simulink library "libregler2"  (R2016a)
settings: Solver=ode45  SolverMode=SingleTasking  StartTime=0.0  StopTime=10.0  RelTol=1e-3
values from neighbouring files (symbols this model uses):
  b0 = 5e3    (= 5000)    [init_epidemie.m]
  g = 9.81    [init_pendelStange.m]
  l = 1    [init_pendelStange.m]    (also in sfun_pendelstangeanim.m = block.DialogPrm(2).Data)
  M = block.DialogPrm(1).Data    [sfun_inferenz.m]
  om0 = 0    [init_pendelStange.m]
  T = 2    [fourierrechteck.m]
undefined symbols (not defined in the file or in its folder): D, h, Kd, Ki, Kp, mk, ml, n, offset, w, x0
libraries: libregler2 x22, simulink x1

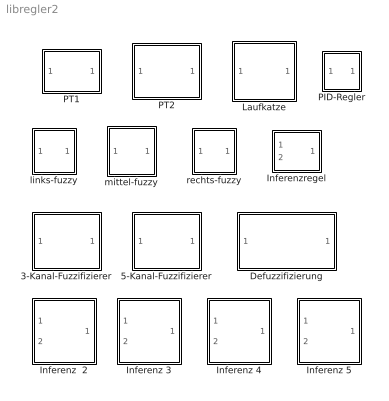
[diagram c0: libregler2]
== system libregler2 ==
  3-Kanal-Fuzzifizierer : Subsystem
  5-Kanal-Fuzzifizierer : Subsystem
  Defuzzifizierung : Subsystem
  Inferenz  2 : Subsystem
  Inferenz 3 : Subsystem
  Inferenz 4 : Subsystem
  Inferenz 5 : Subsystem
  Inferenzregel : Subsystem
  Laufkatze : Subsystem
  PID-Regler : Subsystem
  PT1 : Subsystem
  PT2 : Subsystem
  links-fuzzy : Subsystem
  mittel-fuzzy : Subsystem
  rechts-fuzzy : Subsystem

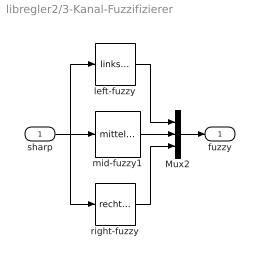
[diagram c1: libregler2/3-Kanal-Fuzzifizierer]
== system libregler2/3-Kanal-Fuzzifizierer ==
  sharp : Inport
  Mux2 : Mux  Inputs=3
  left-fuzzy : libregler2/links-fuzzy  SystemSampleTime=-1  x0=offset-w  w=w
  mid-fuzzy1 : libregler2/mittel-fuzzy  SystemSampleTime=-1  x0=offset  w=w
  right-fuzzy : libregler2/rechts-fuzzy  SystemSampleTime=-1  x0=offset+w  w=w
  fuzzy : Outport
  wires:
  sharp/1 -> right-fuzzy/1, left-fuzzy/1, mid-fuzzy1/1
  Mux2/1 -> fuzzy/1
  mid-fuzzy1/1 -> Mux2/2
  right-fuzzy/1 -> Mux2/3
  left-fuzzy/1 -> Mux2/1

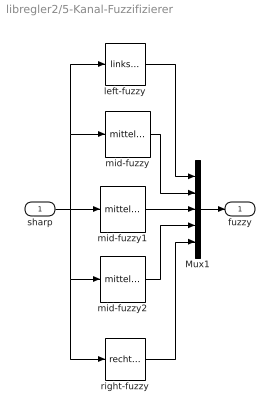
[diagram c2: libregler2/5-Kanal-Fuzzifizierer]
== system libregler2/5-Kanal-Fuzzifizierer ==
  sharp : Inport
  Mux1 : Mux  Inputs=5
  left-fuzzy : libregler2/links-fuzzy  SystemSampleTime=-1  x0=offset-2*w  w=w
  mid-fuzzy : libregler2/mittel-fuzzy  SystemSampleTime=-1  x0=offset-w  w=w
  mid-fuzzy1 : libregler2/mittel-fuzzy  SystemSampleTime=-1  x0=offset  w=w
  mid-fuzzy2 : libregler2/mittel-fuzzy  SystemSampleTime=-1  x0=offset+w  w=w
  right-fuzzy : libregler2/rechts-fuzzy  SystemSampleTime=-1  x0=offset+2*w  w=w
  fuzzy : Outport
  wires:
  Mux1/1 -> fuzzy/1
  sharp/1 -> mid-fuzzy/1, left-fuzzy/1, mid-fuzzy2/1, right-fuzzy/1, mid-fuzzy1/1
  right-fuzzy/1 -> Mux1/5
  mid-fuzzy2/1 -> Mux1/4
  mid-fuzzy1/1 -> Mux1/3
  mid-fuzzy/1 -> Mux1/2
  left-fuzzy/1 -> Mux1/1

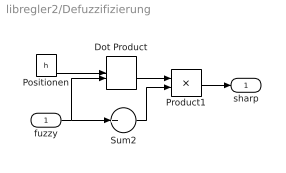
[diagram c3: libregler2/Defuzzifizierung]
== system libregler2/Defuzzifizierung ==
  fuzzy : Inport
  Dot Product : DotProduct
  Positionen : Constant  Value=h
  Product1 : Product  Inputs=*/
  Sum2 : Sum  Inputs=+
  sharp : Outport
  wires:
  Dot Product/1 -> Product1/1
  fuzzy/1 -> Sum2/1, Dot Product/2
  Positionen/1 -> Dot Product/1
  Sum2/1 -> Product1/2
  Product1/1 -> sharp/1

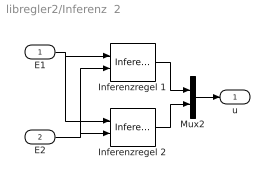
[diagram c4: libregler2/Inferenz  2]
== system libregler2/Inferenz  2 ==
  E1 : Inport
  E2 : Inport  Port=2
  Inferenzregel 1 : libregler2/Inferenzregel  SystemSampleTime=-1  M=M  n=1
  Inferenzregel 2 : libregler2/Inferenzregel  SystemSampleTime=-1  M=M  n=2
  Mux2 : Mux  Inputs=2
  u : Outport
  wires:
  E2/1 -> Inferenzregel 2/2, Inferenzregel 1/2
  E1/1 -> Inferenzregel 2/1, Inferenzregel 1/1
  Inferenzregel 1/1 -> Mux2/1
  Mux2/1 -> u/1
  Inferenzregel 2/1 -> Mux2/2

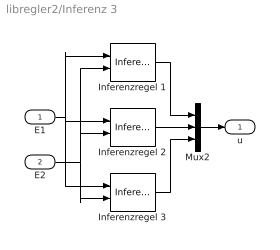
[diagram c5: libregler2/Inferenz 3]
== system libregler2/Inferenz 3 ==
  note: .
  E1 : Inport
  E2 : Inport  Port=2
  Inferenzregel 1 : libregler2/Inferenzregel  SystemSampleTime=-1  M=M  n=1
  Inferenzregel 2 : libregler2/Inferenzregel  SystemSampleTime=-1  M=M  n=2
  Inferenzregel 3 : libregler2/Inferenzregel  SystemSampleTime=-1  M=M  n=3
  Mux2 : Mux  Inputs=3
  u : Outport
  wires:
  E2/1 -> Inferenzregel 3/2, Inferenzregel 1/2, Inferenzregel 2/2
  E1/1 -> Inferenzregel 1/1, Inferenzregel 2/1, Inferenzregel 3/1
  Inferenzregel 3/1 -> Mux2/3
  Inferenzregel 1/1 -> Mux2/1
  Mux2/1 -> u/1
  Inferenzregel 2/1 -> Mux2/2

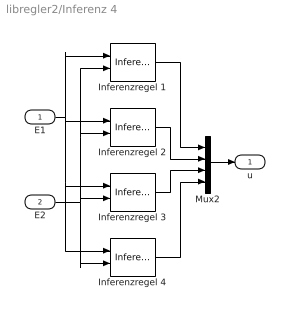
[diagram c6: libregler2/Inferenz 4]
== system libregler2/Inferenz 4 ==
  E1 : Inport
  E2 : Inport  Port=2
  Inferenzregel 1 : libregler2/Inferenzregel  SystemSampleTime=-1  M=M  n=1
  Inferenzregel 2 : libregler2/Inferenzregel  SystemSampleTime=-1  M=M  n=2
  Inferenzregel 3 : libregler2/Inferenzregel  SystemSampleTime=-1  M=M  n=3
  Inferenzregel 4 : libregler2/Inferenzregel  SystemSampleTime=-1  M=M  n=4
  Mux2 : Mux
  u : Outport
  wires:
  E2/1 -> Inferenzregel 2/2, Inferenzregel 1/2, Inferenzregel 3/2, Inferenzregel 4/2
  E1/1 -> Inferenzregel 2/1, Inferenzregel 1/1, Inferenzregel 3/1, Inferenzregel 4/1
  Inferenzregel 3/1 -> Mux2/3
  Inferenzregel 1/1 -> Mux2/1
  Mux2/1 -> u/1
  Inferenzregel 2/1 -> Mux2/2
  Inferenzregel 4/1 -> Mux2/4

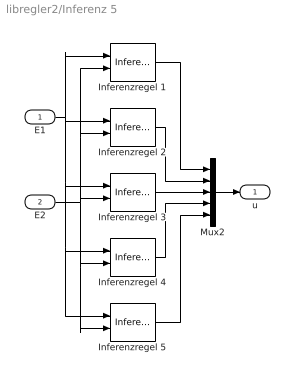
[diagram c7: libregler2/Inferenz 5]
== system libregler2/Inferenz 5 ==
  E1 : Inport
  E2 : Inport  Port=2
  Inferenzregel 1 : libregler2/Inferenzregel  SystemSampleTime=-1  M=M  n=1
  Inferenzregel 2 : libregler2/Inferenzregel  SystemSampleTime=-1  M=M  n=2
  Inferenzregel 3 : libregler2/Inferenzregel  SystemSampleTime=-1  M=M  n=3
  Inferenzregel 4 : libregler2/Inferenzregel  SystemSampleTime=-1  M=M  n=4
  Inferenzregel 5 : libregler2/Inferenzregel  SystemSampleTime=-1  M=M  n=5
  Mux2 : Mux  Inputs=5
  u : Outport
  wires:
  E2/1 -> Inferenzregel 3/2, Inferenzregel 4/2, Inferenzregel 5/2, Inferenzregel 1/2, Inferenzregel 2/2
  E1/1 -> Inferenzregel 3/1, Inferenzregel 4/1, Inferenzregel 5/1, Inferenzregel 1/1, Inferenzregel 2/1
  Inferenzregel 3/1 -> Mux2/3
  Inferenzregel 1/1 -> Mux2/1
  Mux2/1 -> u/1
  Inferenzregel 2/1 -> Mux2/2
  Inferenzregel 4/1 -> Mux2/4
  Inferenzregel 5/1 -> Mux2/5

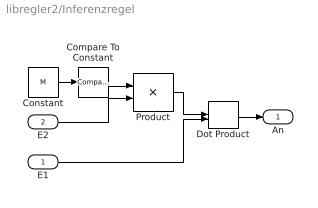
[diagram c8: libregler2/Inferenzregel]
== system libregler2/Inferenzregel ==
  E1 : Inport
  E2 : Inport  Port=2
  Compare To Constant : simulink/Logic and Bit Operations/Compare To Constant  SystemSampleTime=-1  relop===  const=n  LogicOutDataTypeMode=uint8  ZeroCross=off
  Constant : Constant  Value=M
  Dot Product : DotProduct
  Product : Product  Multiplication=Matrix(*)
  An : Outport
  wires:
  Dot Product/1 -> An/1
  E1/1 -> Dot Product/2
  Product/1 -> Dot Product/1
  E2/1 -> Product/2
  Constant/1 -> Compare To Constant/1
  Compare To Constant/1 -> Product/1

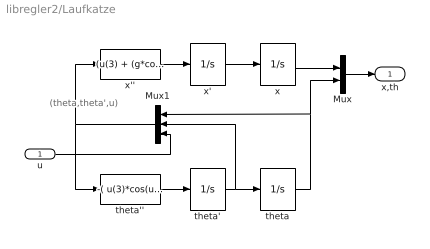
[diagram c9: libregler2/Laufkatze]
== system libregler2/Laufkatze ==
  note: (theta,theta',u)
  u : Inport
  Mux : Mux  Inputs=2
  Mux1 : Mux  Inputs=3
  theta : Integrator
  theta' : Integrator
  theta'' : Fcn  Expr=-( u(3)*cos(u(1)) + (g + l*u(2)^2*cos(u(1)))*ml*sin(u(1)) + g*mk*sin(u(1)) ) / ( (mk + ml*sin(u(1))^2)*l )
  x : Integrator
  x' : Integrator
  x'' : Fcn  Expr=(u(3) + (g*cos(u(1)) + l*u(2)^2)*ml*sin(u(1)))/(mk + ml*sin(u(1))^2)
  x,th : Outport
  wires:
  theta''/1 -> theta'/1
  x''/1 -> x'/1
  u/1 -> Mux1/3
  theta'/1 -> Mux1/2, theta/1
  x'/1 -> x/1
  Mux1/1 -> theta''/1, x''/1
  theta/1 -> Mux1/1, Mux/2
  x/1 -> Mux/1
  Mux/1 -> x,th/1

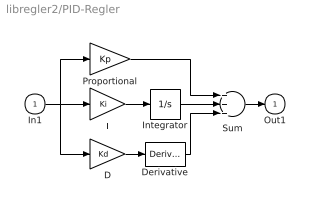
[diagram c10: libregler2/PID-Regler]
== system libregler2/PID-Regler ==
  In1 : Inport
  D : Gain  Gain=Kd
  Derivative : Derivative
  I : Gain  Gain=Ki
  Integrator : Integrator
  Proportional : Gain  Gain=Kp
  Sum : Sum  Inputs=+++
  Out1 : Outport  InitialOutput=0
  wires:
  D/1 -> Derivative/1
  Sum/1 -> Out1/1
  In1/1 -> D/1, Proportional/1, I/1
  Derivative/1 -> Sum/3
  Integrator/1 -> Sum/2
  Proportional/1 -> Sum/1
  I/1 -> Integrator/1

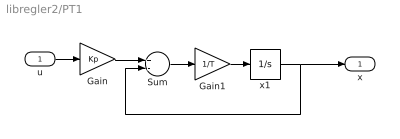
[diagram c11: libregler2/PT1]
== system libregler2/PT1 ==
  u : Inport
  Gain : Gain  Gain=Kp
  Gain1 : Gain  Gain=1/T
  Sum : Sum  Inputs=+-
  x1 : Integrator
  x : Outport
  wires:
  Gain1/1 -> x1/1
  Sum/1 -> Gain1/1
  x1/1 -> Sum/2, x/1
  Gain/1 -> Sum/1
  u/1 -> Gain/1

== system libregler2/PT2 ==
  u : Inport
  Transfer Fcn : TransferFcn  Numerator=[b0]  Denominator=[1 2*D*om0 om0*om0]
  x : Outport
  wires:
  u/1 -> Transfer Fcn/1
  Transfer Fcn/1 -> x/1

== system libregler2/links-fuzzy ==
  In1 : Inport
  Look-Up Table : Lookup  InputValues=[x0 x0+w]  Table=[1 0]  LookUpMeth=Interpolation-Use End Values
  Out1 : Outport
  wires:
  In1/1 -> Look-Up Table/1
  Look-Up Table/1 -> Out1/1

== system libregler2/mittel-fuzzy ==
  In1 : Inport
  Look-Up Table : Lookup  InputValues=[x0-w x0 x0+w]  Table=[0 1 0]  LookUpMeth=Interpolation-Use End Values
  Out1 : Outport
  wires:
  In1/1 -> Look-Up Table/1
  Look-Up Table/1 -> Out1/1

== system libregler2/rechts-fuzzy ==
  In1 : Inport
  Look-Up Table : Lookup  InputValues=[x0-w x0]  Table=[0 1]  LookUpMeth=Interpolation-Use End Values
  Out1 : Outport
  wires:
  In1/1 -> Look-Up Table/1
  Look-Up Table/1 -> Out1/1
